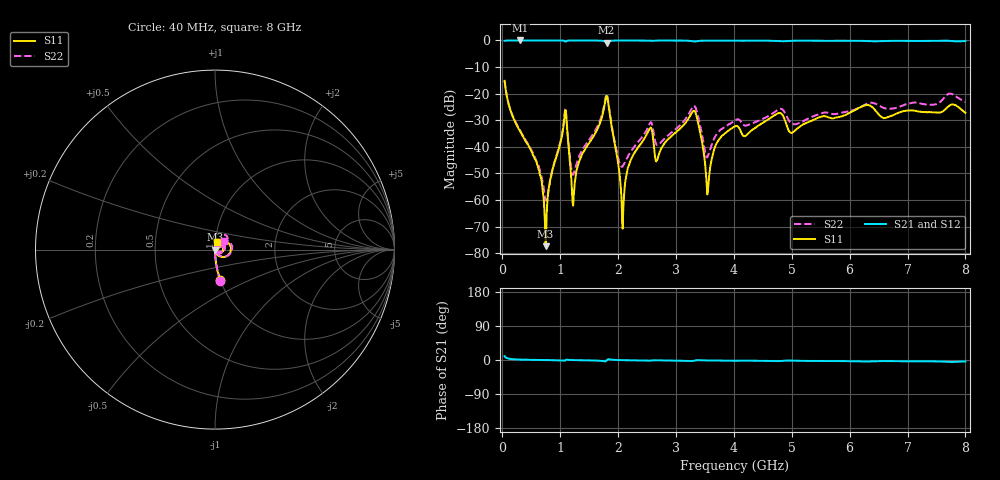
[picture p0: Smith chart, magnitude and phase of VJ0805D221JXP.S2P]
! VJ0805D221JXP
! DATE 03/14/2022  09:05
! CAPACITORS MOUNTED IN SERIES ON 25 MIL THICK MICROSTRIP SUBSTRATE
# GHz  S  MA  R  50.00
!  FREQ  S11M  S11A  S21M  S21A  S12M  S12A  S22M  S22A
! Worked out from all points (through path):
!   801 points, 40 MHz to 8 GHz, reference 50 ohm
!   highest |S21| = 0.00 dB at 308.6 MHz (marker M1); lowest = -0.8 dB at 1.801 GHz (marker M2)
!   lowest |S11| = -77.4 dB at 746.5 MHz (marker M3), VSWR 1.00, Z = 50 + j0.0104 ohm
!   |S11| at or under -10 dB: start of sweep to end of sweep
!   |S22| runs from -60.4 to -15.1 dB; largest |S21 - S12| = 0.0031
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0.04  0.1744 -80.0  0.984 10.1  0.9834 10.1  0.1759 -80.2
0.30865  0.01941 -88.8  1 1.1  0.9995 1.1  0.02034 -88.2
0.6171  0.004223 -89.7  0.9998 0.2  0.9997 0.2  0.004578 -82.8
0.74645  0.0001353 49.9  0.9997 -0.1  1 -0.2  0.001051 -26.2
1.0748  0.03718 48.8  0.9762 -1.9  0.976 -1.9  0.03984 49.9
1.1146  0.02608 -49.2  0.9818 0.9  0.9815 0.9  0.02839 -43.8
1.22405  0.0007857 33.6  0.9986 -0.3  0.9984 -0.3  0.002986 16.3
1.3733  0.007083 86.0  0.9989 -0.7  0.999 -0.7  0.008379 71.7
1.80115  0.09015 7.4  0.908 -1.4  0.908 -1.4  0.09814 11.8
2.00015  0.004966 -81.1  0.9971 -0.1  0.9975 -0.2  0.006379 -37.4
2.07975  0.0002889 48.2  0.998 -0.5  0.9981 -0.5  0.004312 20.5
2.2091  0.005274 87.8  0.9979 -0.8  0.9984 -0.8  0.0078 61.1
2.53745  0.02127 57.4  0.9887 -1.7  0.989 -1.7  0.02599 56.9
2.69665  0.006735 68.0  0.9958 -1.0  0.9961 -1.0  0.01102 45.1
3.31355  0.04745 9.7  0.9566 -1.9  0.9564 -1.9  0.0589 20.1
3.55235  0.001568 166.9  0.9896 -1.3  0.9899 -1.3  0.006716 37.3
3.71155  0.01205 103.5  0.9908 -1.4  0.991 -1.5  0.01784 70.7
4.02995  0.02445 70.0  0.9879 -2.1  0.9879 -2.1  0.0319 57.7
5.3533  0.03127 76.1  0.9888 -2.6  0.9887 -2.6  0.03692 58.8
6.29855  0.06131 67.3  0.9739 -4.0  0.9741 -4.1  0.06466 53.6
6.67665  0.0367 76.4  0.9808 -3.0  0.9809 -3.0  0.05192 43.0
8  0.04368 72.8  0.9722 -3.7  0.9726 -3.8  0.07017 43.0
